PROGRAM MAIN
// Variable declaration example program 5
VAR CONSTANT
   NumOfFilterCoeff               :BYTE:=40;
END_VAR
VAR
   // Function block "Tc2_EtherCAT" for CoE Object access:
   fb_coe_write                   :FB_EcCoESdoWrite;
   userNetId                      :T_AmsNetId := 'xxx.xx.1.1.2.1';
   userSlaveAddr                  :UINT := 1001;
   // Status zur Übertragung der Filter-Koeffizienten (Set to 0 for start)
   wState                         :BYTE:=255;
   index                          :BYTE:=1; // Index for coefficients transfer
   wCoEIndexUserFilterCoeffizents :WORD:=16#8001;
   aFilterCoeffs:ARRAY[0..NumOfFilterCoeff] OF LREAL :=
   [// Example filter coefficients band pass: 3600..3900 Hz
      0.03663651655662163,
      0.04299467480848277,
      -0.007880289104928245,
      0.0664029021294729,
      -0.0729038234874446,
      -0.00005849791174519834,
      0.05628409460964408,
      -0.0525134329294473,
      0.026329003448584205,
      0.00027114381194760643,
      -0.03677629552114248,
      0.06743018479714939,
      -0.0560894442193289,
      0.0009722394088121363,
      0.05676876756757213,
      -0.07775650809213645,
      0.05330627422911416,
      0.0009941073749156226,
      -0.055674804078696793,
      0.07874009379691002,
      -0.055674804078696793,
      0.0009941073749156226,
      0.05330627422911416,
      -0.07775650809213645,
      0.05676876756757213,
      0.0009722394088121363,
      -0.0560894442193289,
      0.06743018479714939,
      -0.03677629552114248,
      0.00027114381194760643,
      0.026329003448584205,
      -0.0525134329294473,
      0.05628409460964408,
      -0.00005849791174519834,
      -0.0729038234874446,
      0.0664029021294729,
      -0.007880289104928245,
      0.04299467480848277,
      0.03663651655662163,
      0
   ];
   nValue                     :DINT; // Temporary variable
END_VAR

// Example program 5:
// writes filter coefficients of
// "User defined FIR Filter" (32)
// incl. example coefficients for band pass
// Note: writing possible, if CoE Object
// PAI Settings Ch.1 (0x8000:16) has value 32 or 33 set, only!
// (32 = User defined FIR Filter / 33 = User defined IIR Filter)
// ===============================================================
CASE wState OF
   0:
      fb_coe_write(bExecute := FALSE);// Prepare CoE access
      wState := wState + 1;// Go to next state
   1:
      //nValue := REAL_TO_DINT(DINT_TO_REAL(aFilterCoeffs[index]) *16384);
      nValue := LREAL_TO_DINT(aFilterCoeffs[index] * 1073741824); // Bit-shift factor: 2^30
      // Write filter coefficients (max. 40 entries)
      fb_coe_write(
      sNetId:= userNetId,
      nSlaveAddr:= userSlaveAddr,
      nSubIndex:= index,
      nIndex:= wCoEIndexUserFilterCoeffizents,
      pSrcBuf:= ADR(nValue),
      cbBufLen:= SIZEOF(nValue),
      bExecute:= TRUE,
      tTimeout:= T#1S
      );
      wState := wState + 1; // Go to next state
   2:
      // Execute writing to CoE
      fb_coe_write();
      IF fb_coe_write.bError THEN
         wState := 100; // Error case
      ELSE
         IF NOT fb_coe_write.bBusy THEN
            index := index + 1;
            IF index <= (NumOfFilterCoeff) THEN
               fb_coe_write(bExecute := FALSE);// Prepare the next CoE access
               wState := 1;// Nächsten Wert Schreiben
            ELSE
               wState := 255;// Done
            END_IF
         END_IF
      END_IF
   100:
      ; // Error handling
   255:
      ; // End
END_CASE

END_PROGRAM
